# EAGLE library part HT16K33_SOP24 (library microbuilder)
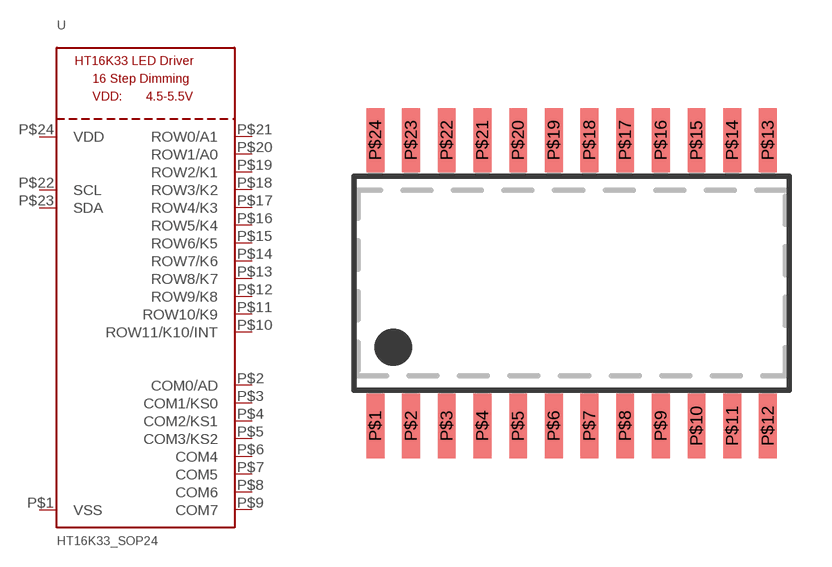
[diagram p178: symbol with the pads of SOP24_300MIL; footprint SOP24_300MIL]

Designator prefix U

## HT16K33_SOP24  [SOP24_300MIL]
P$1  VSS
P$2  COM0/AD
P$3  COM1/KS0
P$4  COM2/KS1
P$5  COM3/KS2
P$6  COM4
P$7  COM5
P$8  COM6
P$9  COM7
P$10  ROW11/K10/INT
P$11  ROW10/K9
P$12  ROW9/K8
P$13  ROW8/K7
P$14  ROW7/K6
P$15  ROW6/K5
P$16  ROW5/K4
P$17  ROW4/K3
P$18  ROW3/K2
P$19  ROW2/K1
P$20  ROW1/A0
P$21  ROW0/A1
P$22  SCL
P$23  SDA
P$24  VDD

## Footprint SOP24_300MIL (pad centres in mm)
smd 0.635 x 2.286: P$1 -6.985,-5.08; P$2 -5.715,-5.08; P$3 -4.445,-5.08; P$4 -3.175,-5.08; P$5 -1.905,-5.08; P$6 -0.635,-5.08; P$7 0.635,-5.08; P$8 1.905,-5.08; P$9 3.175,-5.08; P$10 4.445,-5.08; P$11 5.715,-5.08; P$12 6.985,-5.08; P$13 6.985,5.08; P$14 5.715,5.08; P$15 4.445,5.08; P$16 3.175,5.08; P$17 1.905,5.08; P$18 0.635,5.08; P$19 -0.635,5.08; P$20 -1.905,5.08; P$21 -3.175,5.08; P$22 -4.445,5.08; P$23 -5.715,5.08; P$24 -6.985,5.08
